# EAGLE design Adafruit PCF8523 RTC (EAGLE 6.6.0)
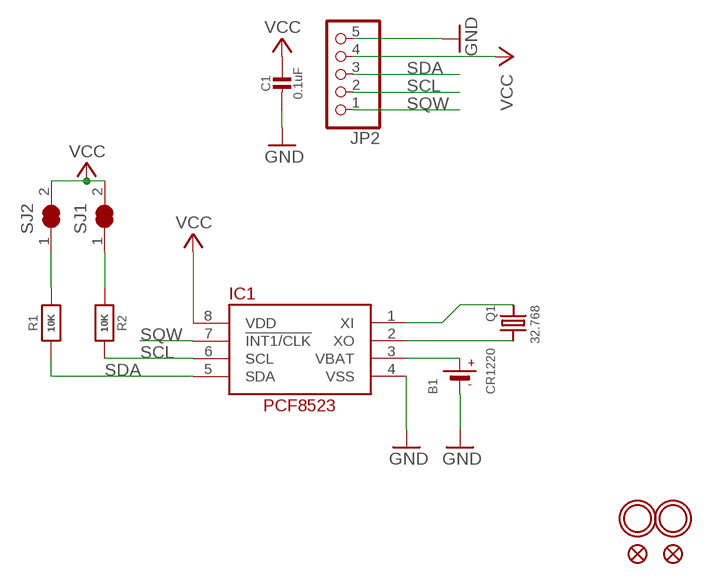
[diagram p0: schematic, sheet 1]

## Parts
B1  CR1220  BATTERYCR1220_SMT  [CR1220]
C1  0.1uF  CAP_CERAMIC0805-NOOUTLINE  [0805-NO]
FID1  FIDUCIAL""  [FIDUCIAL_1MM]
FID2  FIDUCIAL""  [FIDUCIAL_1MM]
IC1  RTC_PCF8523T  [SOIC8_150MIL]
JP2  HEADER-1X576MIL  [1X05_ROUND_76]
Q1  32.768  CRYSTAL8.0X3.8  [CRYSTAL_8X3.8]
R1  10K  RESISTOR0805_NOOUTLINE  [0805-NO]
R2  10K  RESISTOR0805_NOOUTLINE  [0805-NO]
SJ1  SOLDERJUMPER_CLOSED  [SOLDERJUMPER_CLOSEDWIRE]
SJ2  SOLDERJUMPER_CLOSED  [SOLDERJUMPER_CLOSEDWIRE]
U$1  MOUNTINGHOLE2.0  [MOUNTINGHOLE_2.0_PLATED]
U$4  MOUNTINGHOLE2.0  [MOUNTINGHOLE_2.0_PLATED]

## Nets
GND: B1.- C1.2 IC1.4(VSS) JP2.5
N$1: R2.1 SJ1.1
N$2: R1.2 SJ2.1
N$14: IC1.1(XI) Q1.P$1
N$15: IC1.2(XO) Q1.P$4
SCL: IC1.6(SCL) JP2.2 R2.2
SDA: IC1.5(SDA) JP2.3 R1.1
SQW: IC1.7(!INT1/CLK) JP2.1
VBAT: B1.+$1(+) IC1.3(VBAT)
VCC: C1.1 IC1.8(VDD) JP2.4 SJ1.2 SJ2.2

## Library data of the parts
B1 = microbuilder:BATTERY: CR1220 SMT - Digikey: 3001K-ND
C1 = microbuilder:CAP_CERAMIC: Ceramic Capacitors
FID1 FID2 = microbuilder:FIDUCIAL: Fiducial Alignment Points; BOM: EXCLUDE
IC1 = microbuilder:RTC_PCF8523
JP2 = microbuilder:HEADER-1X5: PIN HEADER
Q1 = microbuilder:CRYSTAL: Crystals
R1 R2 = microbuilder:RESISTOR: Resistors
SJ1 SJ2 = microbuilder:SOLDERJUMPER_CLOSED: Solder Jumper - Closed
U$1 U$4 = microbuilder:MOUNTINGHOLE: Mounting Hole; BOM: EXCLUDE

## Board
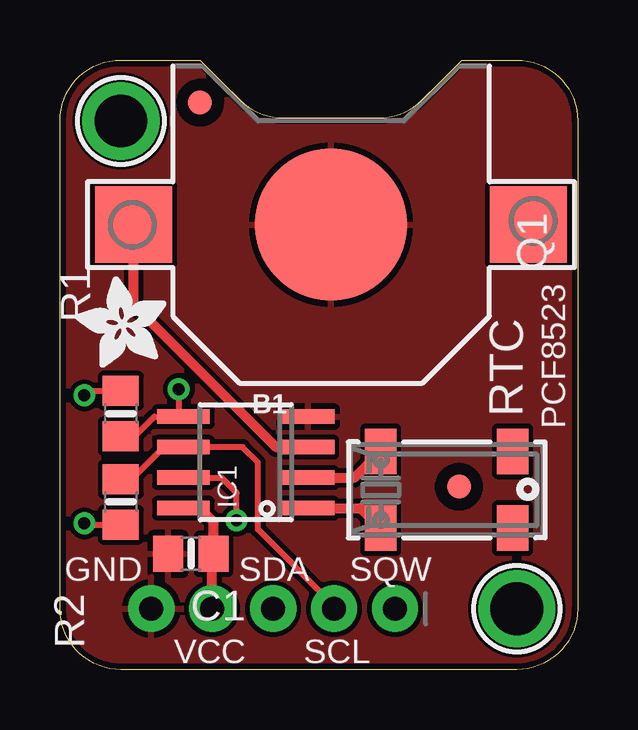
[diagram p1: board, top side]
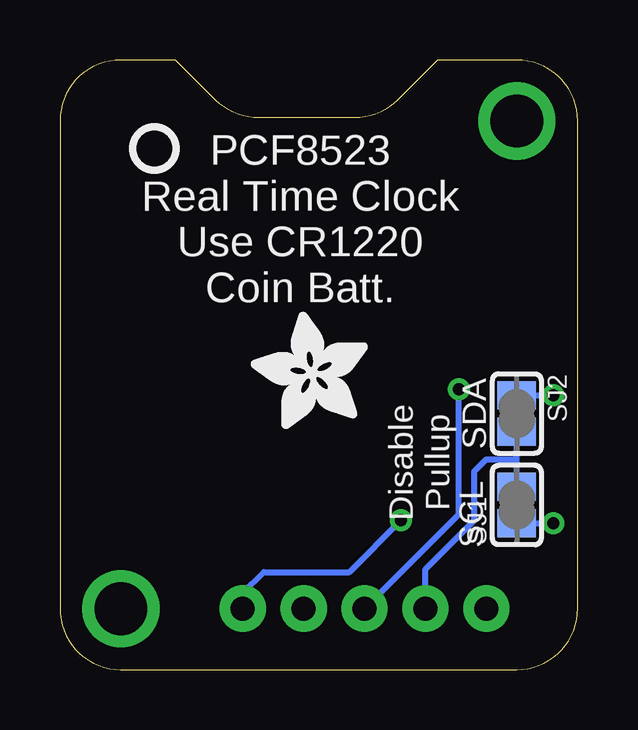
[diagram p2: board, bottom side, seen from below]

Size 21.59 x 25.4 mm. Coordinates in mm from the lower left corner, seen from the top.
Outline: 16.76,25.4 19.05,25.4 arc-90 21.59,22.86 21.59,2.54 arc-90 19.05,0 2.54,0 arc-90 0,2.54 0,22.86 arc-90 2.54,25.4 5.84,25.4 7.51,23.73 arc45 9.31,22.99 13.3,22.99 arc45 15.1,23.73 16.76,25.4
Copper layers (1*16): Top 0.035mm / dielectric 1.5mm / Bottom 0.035mm
Design rules "adafruit *": minimum track width 8mil, minimum drill 15.5mil, track to track 8mil, track to pad 8mil, pad to pad 8mil, via to via 8mil, smd to smd 8mil, copper to edge 10mil, drill to drill 8mil, minimum pad ring 10mil, minimum via ring 8mil, stop-mask expansion 2mil, vias tented up to drill 20mil, thermal gap 10mil

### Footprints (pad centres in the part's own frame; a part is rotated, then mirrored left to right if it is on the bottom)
CR1220 = smd 3.2 x 3.2: +$1 -8.225,0; +$2 8.225,0 | smd 6.35 x 6.35: - 0,0
0805-NO = smd 1.24 x 1.5: 1 -0.95,0; 2 0.95,0
FIDUCIAL_1MM = smd 1 x 1: 1 0,0
SOIC8_150MIL = smd 0.6 x 2.2: 1 -1.905,-2.6; 2 -0.635,-2.6; 3 0.635,-2.6; 4 1.905,-2.6; 5 1.905,2.6; 6 0.635,2.6; 7 -0.635,2.6; 8 -1.905,2.6
1X05_ROUND_76 = drill 1 pad 1.93: 1 -5.08,0; 2 -2.54,0; 3 0,0; 4 2.54,0; 5 5.08,0
CRYSTAL_8X3.8 = smd 1.3 x 1.9: P$1 -2.75,-1.6; P$2 2.75,-1.6; P$3 2.75,1.6; P$4 -2.75,1.6
SOLDERJUMPER_CLOSEDWIRE = smd 1.168 x 1.6: 1 -0.762,0; 2 0.762,0 | smd 0.635 x 0.203: WIRE 0,0
MOUNTINGHOLE_2.0_PLATED = drill 2.2 pad 3: P$1 0,0

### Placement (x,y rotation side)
B1  11.3,18.54 0 top
C1  5.46,4.83 180 top
FID1  5.84,23.62 90 top
FID2  16.64,7.62 90 top
IC1  7.75,8.64 90 top
JP2  8.89,2.54 180 top
Q1  16.13,7.49 0 top
R1  2.54,10.67 90 top
R2  2.54,6.99 90 top
SJ1  2.54,6.86 90 bottom
SJ2  2.54,10.67 270 bottom
U$1  2.54,22.86 90 top
U$2  [ADAFRUIT_3.5MM]  4.45,12.57 90 top
U$3  [PCBFEAT-REV-040]  17.65,21.72 180 bottom
U$4  19.05,2.54 90 top
U$5  [ADAFRUIT_5MM]  8.76,10.03 90 bottom

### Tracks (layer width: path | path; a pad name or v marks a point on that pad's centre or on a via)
GND
  pour Top: 0,0 21.59,0 21.59,25.4 0,25.4
N$1  (via drill 0.5)
  Top 0.254: v1.02,6.1 1.08,6.04 R2.1
  Bottom 0.254: SJ1.1 v1.02,6.1
N$2  (via drill 0.5)
  Top 0.254: v1.02,11.43 1.2,11.62 R1.2
  Bottom 0.254: SJ2.1 v1.02,11.43
N$14
  Top 0.406: IC1.1 12.54,6.73 Q1.P$1
N$15
  Top 0.406: IC1.2 12.29,8 Q1.P$4
SCL
  Top 0.254: JP2.2 11.43,2.67 8.26,5.84 8.26,8.64 7.62,9.27 IC1.6 4.32,9.27 2.98,7.93 R2.2
SDA  (via drill 0.5)
  Top 0.254: v4.95,11.68 4.95,10.73 IC1.5 3.94,10.54 3.11,9.72 R1.1
  Bottom 0.254: JP2.3 4.95,6.48 v4.95,11.68
SQW  (via drill 0.5)
  Top 0.254: v7.37,6.22 7.37,7.37 6.73,8 IC1.7
  Bottom 0.254: JP2.1 13.97,3.17 13.08,4.06 9.53,4.06 v7.37,6.22
VBAT
  Top 0.406: B1.+$1 3.08,15.21 9.02,9.27 IC1.3
VCC
  Top 0.406: IC1.8 5.84,6.73 6.41,6.16 C1.1 6.35,4.76 JP2.4
  Bottom 0.254: SJ1.2 2.54,8.76 | 2.54,8.76 SJ2.2 | JP2.4 6.35,4.19 4.32,6.22 4.32,8.26 3.81,8.76 2.54,8.76

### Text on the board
tPlace: RTC | PCF8523 | GND | SDA | SQW | VCC | SCL
bPlace: PCF8523 / Real Time Clock / Use CR1220 / Coin Batt. | SDA | Disable / Pullup | SCL

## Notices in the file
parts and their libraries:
microbuilder: This work is placed in the public domain, and may be freely used for commercial and non-commercial work with the following conditions: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
